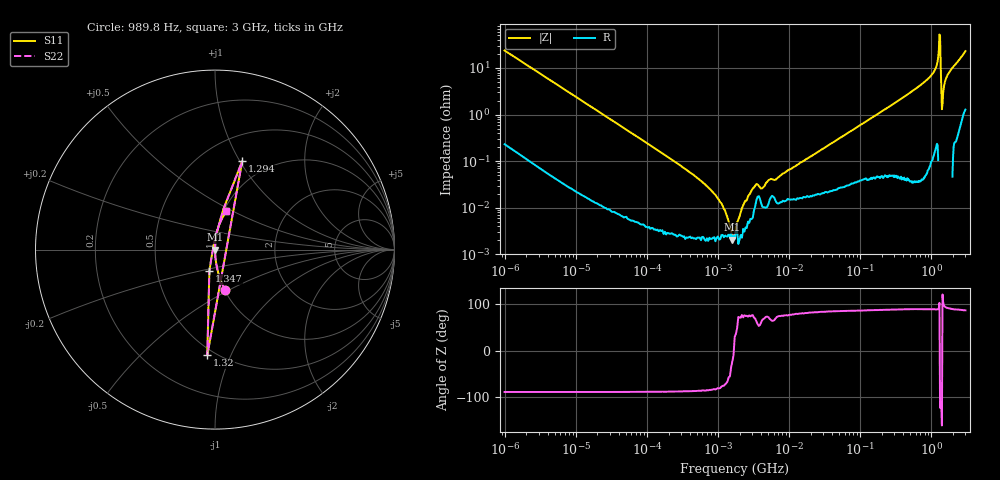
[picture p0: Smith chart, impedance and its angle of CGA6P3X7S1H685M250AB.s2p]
! S-Parameter Data Generated by TDK Corporation
! Copyright(C) 2020 TDK Corporation.
! All Rights Reserved.
! TDK P/N: CGA6P3X7S1H685M250AB (Multilayer Ceramic Chip Capacitor)
! Property: C=6.8uF
! Size(LxWxT): 3.2x2.5x2.5mm
! Model Type: s2p (Touchstone File Format Version 1.0)
! Frequency: DC=Yes Start=0.000989846MHz Stop=3000MHz 463points Log-sweep
! Model Generated on Aug. 18, 2020
! Port Assignments:
!  1 ---| |--- 2
! Applicable Conditions:
!  Temperature = 25 degC
!  DC Bias Voltage = 0 V
!  Small Signal Operation
! Terms and conditions regarding TDK Simulation Models
! (1)This simulation model is being provided solely for informational purposes. Please refer to the specifications of the products in terms of detailed characteristics of such products.
! (2)In no event shall TDK Corporation of any of its subsidiaries be liable for any loss or damage arising, directly or indirectly,
!  From any information contained in this simulation model, including, but not limited to loss or damages arising from any inaccuracies, omissions or errors in connection with such information.
! (3)Any and all copyrights on this simulation model are owned by TDK Corporation.
!  Duplication or redistribution of this simulation model without prior written permission from TDK Corporation is prohibited.
! (4)This simulation model is subject to any modification or change without any prior notice.
! (5)Neither TDK Corporation nor any of its subsidiaries shall make any warranty, express or implied,
!  Including but not limited to the correctness, implied warranties of merchantability and fitness for a particular purpose with respect to this simulation models.
! (6)The use of this simulation model shall be deemed to have consented to the terms and conditions hereof.
# Hz S MA R 50
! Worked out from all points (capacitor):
!   462 points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, 989.8 Hz to 3 GHz, reference 50 ohm
!   read as one part in series: C = 6.75 uF near 1.07 kHz
!   lowest |Z| = 2.08 mohm at 1.578 MHz (marker M1)
!   series resonance near 1.661 MHz, so ESL is about 1.4 nH
!   S11 on the Smith chart (normalised r, x): 989.8 Hz: 1.00, -0.48; 1.294 GHz: 0.76, +1.02; 1.32 GHz: 0.45, -0.82; 1.347 GHz: 0.91, -0.22; 3 GHz: 1.03, +0.46
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989.846  0.2306 -76.1  0.9708 13.3  0.9708 13.3  0.2306 -76.1
12024.64  0.02 -88.3  0.9996 1.1  0.9996 1.1  0.02 -88.3
146075.1  0.001662 -88.8  1 0.1  1 0.1  0.001662 -88.8
595127.2  0.0003611 -86.2  1 0.0  1 0.0  0.0003611 -86.2
1201231  9.547e-05 -75.8  1 0.0  1 0.0  9.547e-05 -75.8
1578499  2.085e-05 -24.2  1 0.0  1 0.0  2.085e-05 -24.2
1774518  3.936e-05 36.2  1 -0.0  1 -0.0  3.936e-05 36.2
2156787  9.874e-05 76.6  1 -0.0  1 -0.0  9.874e-05 76.6
3312886  0.0002968 68.9  0.9999 -0.0  0.9999 -0.0  0.0002968 68.9
4186766  0.0002641 66.6  0.9999 -0.0  0.9999 -0.0  0.0002641 66.6
2.073191e7  0.001306 82.2  0.9998 -0.1  0.9998 -0.1  0.001306 82.2
2.507343e8  0.01463 87.3  0.9994 -0.8  0.9994 -0.8  0.01463 87.3
9.779672e8  0.06732 85.4  0.9968 -3.9  0.9968 -3.9  0.06732 85.4
1.171007e9  0.1077 82.7  0.9921 -6.2  0.9921 -6.2  0.1077 82.7
1.243477e9  0.167 80.0  0.9849 -9.6  0.9849 -9.6  0.167 80.0
1.294266e9  0.5153 72.9  0.9809 -30.1  0.9809 -30.1  0.5153 72.9
1.320433e9  0.59 -94.2  1.198 29.4  1.198 29.4  0.59 -94.2
1.347129e9  0.1228 -104.8  1.038 6.6  1.038 6.6  0.1228 -104.8
1.402151e9  0.01325 -161.5  1.013 0.2  1.013 0.2  0.01325 -161.5
1.45942e9  0.02879 102.5  1.007 -1.6  1.007 -1.6  0.02879 102.5
1.67892e9  0.07007 87.9  0.9999 -4.0  0.9999 -4.0  0.07007 87.9
3e9  0.2216 74.0  0.9629 -12.8  0.9629 -12.8  0.2216 74.0
